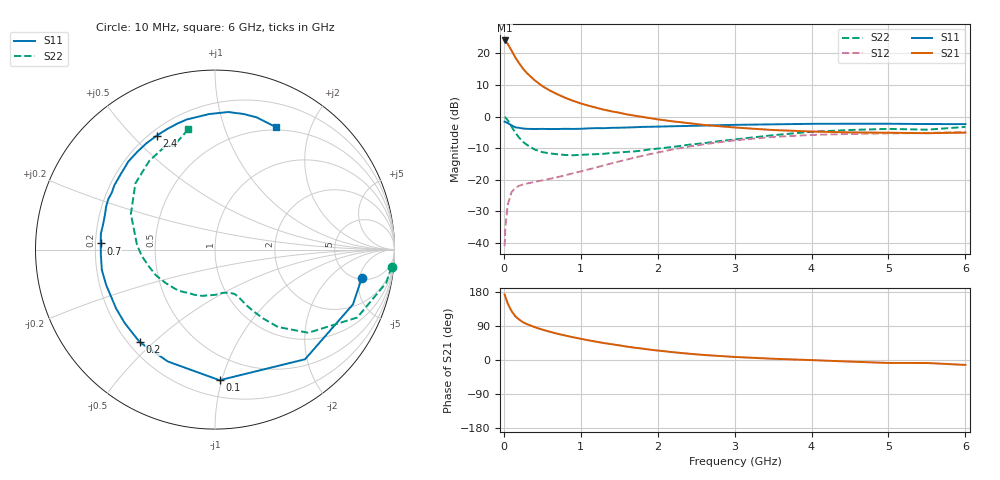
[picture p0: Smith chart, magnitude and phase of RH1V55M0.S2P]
! SIEMENS Small Signal Semiconductors
! BFR106
! Si NPN RF Bipolar Junction Transistor in SOT23
! VCE = 1.5 V  IC = 5 mA
! Common Emitter S-Parameters:  August  1996
# GHz  S  MA  R  50
!  f  S11  S21  S12  S22
! GHz  MAG  ANG  MAG  ANG  MAG  ANG  MAG  ANG
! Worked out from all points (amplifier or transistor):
!   36 points, 10 MHz to 6 GHz, reference 50 ohm
!   highest |S21| = 24.1 dB at 10 MHz (marker M1)
!   |S21| within 3 dB of that: start of sweep to 95.37 MHz
!   unconditionally stable (mu >= 1): 599.8 MHz to 2.419 GHz; 3.983 GHz to end of sweep
!   at 250 MHz: K = 0.51, MSG = 18.3 dB, |S12| = -21.5 dB
!   at 1.4 GHz: K = 1.18, MAG = 5.7 dB, |S12| = -14.8 dB
!   at 6 GHz: K = 1.03, MAG = -1.1 dB, |S12| = -4.8 dB
!   S11 on the Smith chart (normalised r, x): 10 MHz: 5.33, -5.45; 100 MHz: 0.32, -0.98; 200 MHz: 0.24, -0.45; 700 MHz: 0.22, +0.03; 2.4 GHz: 0.23, +0.59; 6 GHz: 0.46, +1.51
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0.01  0.8334 -10.8  16.09 172.8  0.0089 86.0  0.9883 -5.6
0.02  0.8271 -21.6  15.87 167.1  0.0176 81.8  0.9717 -11.0
0.05  0.7907 -50.6  14.21 149.3  0.0401 64.6  0.8784 -25.5
0.1  0.7282 -88.0  11.13 129.1  0.0637 49.2  0.6966 -41.7
0.15  0.6765 -112.8  8.632 115.2  0.075 40.3  0.5555 -50.9
0.2  0.6647 -129.1  6.981 106.5  0.0804 36.5  0.4636 -55.3
0.25  0.6486 -140.9  5.747 99.5  0.0846 34.5  0.3975 -58.4
0.3  0.6413 -149.2  4.891 94.7  0.0874 34.4  0.3583 -60.4
0.4  0.6375 -161.8  3.777 86.8  0.0926 35.2  0.3023 -63.2
0.5  0.6405 -169.9  3.05 80.2  0.0979 37.2  0.2744 -65.5
0.6  0.6365 -177.2  2.583 74.4  0.1039 39.8  0.2615 -68.5
0.7  0.6378 176.9  2.251 69.1  0.1103 42.5  0.2537 -72.5
0.9  0.639 167.3  1.781 60.1  0.1268 47.4  0.2447 -80.2
1.1  0.6522 158.4  1.492 52.0  0.146 51.0  0.2519 -89.8
1.3  0.6566 151.1  1.288 44.8  0.1693 53.2  0.2581 -99.4
1.6  0.6733 141.0  1.086 35.3  0.2092 54.4  0.2771 -114.9
2.2  0.7049 122.9  0.842 20.6  0.3029 50.0  0.3317 -145.7
2.4  0.713 117.1  0.79 16.7  0.3348 47.3  0.3587 -156.4
3.5  0.7557 92.6  0.614 3.3  0.4777 27.6  0.5088 157.1
4.5  0.7721 78.1  0.563 -4.2  0.5323 10.2  0.615 126.6
5.5  0.7638 67.1  0.547 -7.9  0.5515 0.1  0.6219 111.7
6  0.7623 63.6  0.559 -13.0  0.574 -7.1  0.6878 102.4
